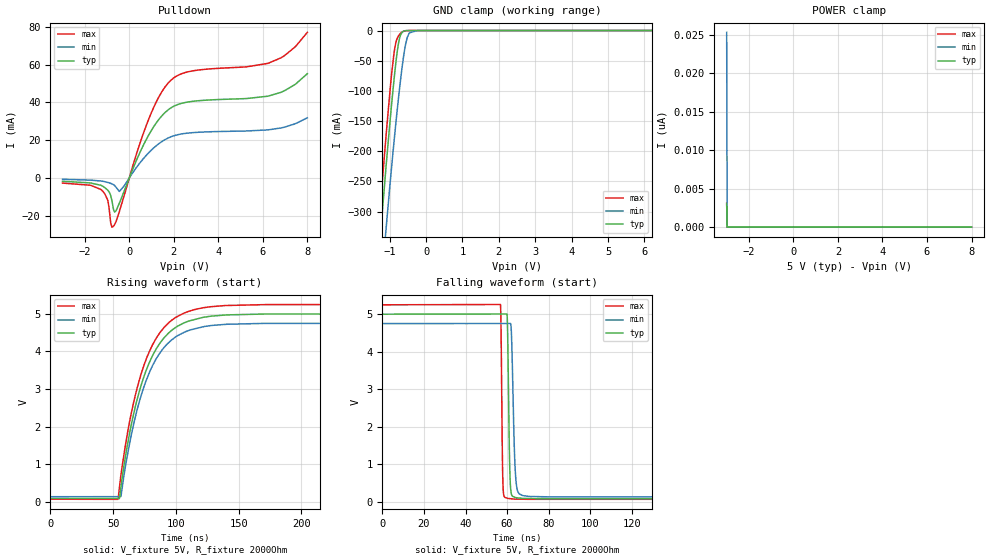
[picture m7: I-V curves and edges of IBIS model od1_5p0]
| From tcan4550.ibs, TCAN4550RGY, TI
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|   od1_5p0 Model
[Model]   od1_5p0
Model_type   Open_drain
Polarity   Non-Inverting
Vmeas = 2.5
Vref = 5
Cref = 2pF
Rref = 2000
|   typ   min   max
C_comp   5.491pF   5.196pF   5.645pF
|  Where Nom  PVT is Nominal Process, 5V,   27C
|   Fast PVT is Strong Process,  5.25, -40C
|   Slow PVT is Weak Process,   4.75V, 150C
[Voltage Range]   5   4.75   5.25
|Junction Temperature
[Temperature Range]   27   150   -40
[Pullup Reference]   5   4.75   5.25
[Pulldown Reference]   0   0   0
[Power Clamp Reference]   5   4.75   5.25
[GND Clamp Reference]   0   0   0
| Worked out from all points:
|   slope of the pulldown table from 0 to 0.75 V, typ, clamps not added: 37.4 ohm
|   GND clamp passes 1 mA (typ) near -0.61 V on its own axis
|   falling waveform, V_fixture 5V, R_fixture 2000Ohm: 20-80 % time 794ps typ, 1.29ns min, 591ps max; typ from 5 V to 0.081 V
|   rising waveform, V_fixture 5V, R_fixture 2000Ohm: 20-80 % time 24.3ns typ, 24.3ns min, 24.1ns max; typ from 0.081 V to 5 V
[Pulldown]
|   Voltage   I(typ)   I(min)   I(max)
-3V       -1.777mA   -713.2uA   -2.735mA
-1.273V   -3.9mA     -1.629mA   -6.126mA
-976mV    -6.396mA   -2.36mA    -11.56mA
-767mV    -12.96mA   -3.217mA   -26.09mA
-591mV    -17.32mA   -4.962mA   -22.99mA
-448mV    -13.44mA   -7.171mA   -17.87mA
861mV     22.48mA    13.2mA     30.79mA
1.818V    36.71mA    21.53mA    51.17mA
2.841V    40.58mA    23.99mA    56.71mA
6.229V    43.31mA    25.45mA    60.69mA
6.966V    46.16mA    26.89mA    64.75mA
8V        55.25mA    31.86mA    77.16mA
[GND Clamp]
|   Voltage   I(typ)   I(min)   I(max)
-3V       -1.786A    -1.824A    -1.778A
-1.537V   -564mA     -654.9mA   -520.7mA
-1.273V   -354.8mA   -454.8mA   -305.7mA
-1.229V   -321.3mA   -422.5mA   -271.5mA
-1.097V   -224.3mA   -327.8mA   -173.2mA
-965mV    -134.5mA   -238.4mA   -83.89mA
-877mV    -79.99mA   -182.6mA   -36.09mA
-745mV    -17.59mA   -105.5mA   -7.944mA
-613mV    -980.8uA   -41.19mA   -1.041mA
-459mV    -19.65uA   -3.879mA   -16.69uA
-239mV    0A         -15.12uA   0A
8V        0A         0A         0A
[POWER Clamp]
|   Voltage   I(typ)   I(min)   I(max)
-3V       3.007nA    25.32nA    3.121nA
-2.978V   0A         0A         0A
-2.967V   0A         0A         0A
8V        0A         0A         0A
[Ramp]
R_load = 2000
|   typ   min   max
dV/dt_r   2.95131/2.43426e-08   2.77216/2.43316e-08   3.11187/2.41019e-08
dV/dt_f   2.95131/7.92991e-10   2.77216/1.28335e-09   3.11187/5.89921e-10
[Falling Waveform]
V_fixture = 5V
V_fixture_min = 4.75V
V_fixture_max = 5.25V
R_fixture = 2000Ohm
C_fixture = 0F
|   Time   V(typ)   V(min)   V(max)
0s        5V         4.75V      5.25V
56.78ns   5.005V     4.752V     5.258V
57.78ns   5.005V     4.752V     1.023V
58.31ns   5.005V     4.752V     200.2mV
60.07ns   4.907V     4.752V     92.94mV
61.2ns    1.064V     4.752V     82.37mV
61.93ns   239.6mV    4.642V     78.68mV
64.27ns   108mV      555.9mV    69.38mV
70.34ns   85.93mV    143.6mV    64.14mV
25us      81.15mV    129.7mV    63.54mV
[Rising Waveform]
V_fixture = 5V
V_fixture_min = 4.75V
V_fixture_max = 5.25V
R_fixture = 2000Ohm
C_fixture = 0F
|   Time   V(typ)   V(min)   V(max)
0s        81.15mV    129.7mV    63.54mV
53.91ns   80.02mV    131.5mV    60.32mV
56.31ns   393.2mV    151.9mV    716.9mV
61.98ns   1.605V     1.339V     1.918V
71.55ns   3.006V     2.734V     3.313V
81.54ns   3.892V     3.629V     4.181V
94.32ns   4.493V     4.235V     4.764V
123ns     4.915V     4.666V     5.169V
172ns     4.997V     4.747V     5.247V
25us      5V         4.75V      5.25V
